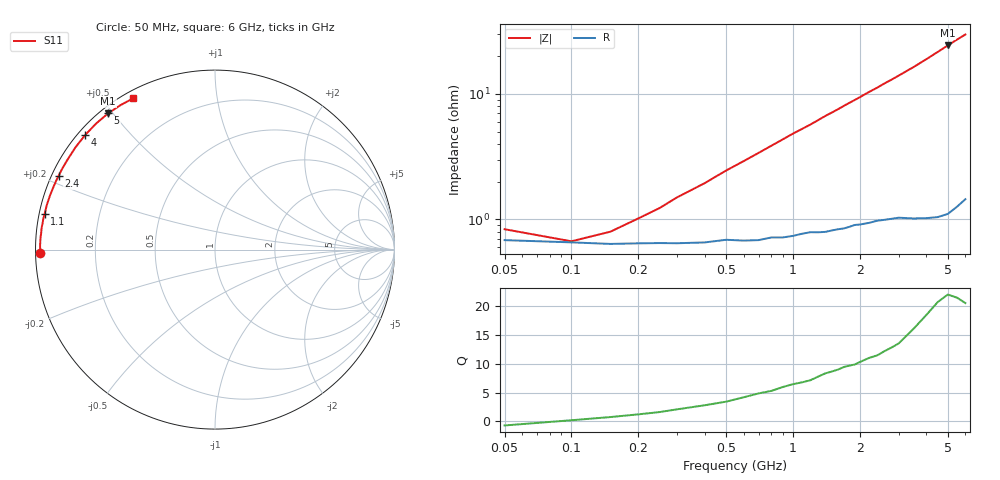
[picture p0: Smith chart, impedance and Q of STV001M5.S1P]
! SIEMENS Discrete & RF Semiconductors
! BA892
! Si PIN Diode in SCD-80
! IF = 1.5 mA
! S-Parameters:  September  1997
# GHz  S  MA  R  50
!  f  S11
! GHz  MAG  ANG
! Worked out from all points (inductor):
!   34 points, 50 MHz to 6 GHz, reference 50 ohm
!   read as one part to ground: L = 755 pH near 500 MHz
!   highest Q = 21.4 at 5 GHz (marker M1), where L = 774 pH
!   S11 on the Smith chart (normalised r, x): 50 MHz: 0.01, -0.01; 1.1 GHz: 0.02, +0.10; 2.4 GHz: 0.02, +0.22; 4 GHz: 0.02, +0.38; 5 GHz: 0.02, +0.49; 6 GHz: 0.03, +0.59
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0.05  0.973 -178.9
0.1  0.9741 179.7
0.15  0.9748 178.9
0.2  0.9745 178.2
0.25  0.9744 177.6
0.3  0.9745 176.9
0.4  0.9741 175.8
0.5  0.9729 174.6
0.7  0.9731 172.4
0.8  0.9718 171.3
1  0.9711 169.1
1.1  0.97 168.1
1.2  0.9692 167.1
1.4  0.9692 164.9
1.6  0.9678 162.9
1.7  0.9675 161.8
2  0.9654 158.8
2.2  0.9646 156.7
2.4  0.9635 154.8
2.6  0.9631 152.7
2.8  0.9627 150.8
3  0.9624 148.8
3.5  0.9639 143.8
4  0.9648 138.6
4.5  0.9654 133.3
5  0.9648 128.1
5.5  0.9617 123.1
6  0.9581 118.5
